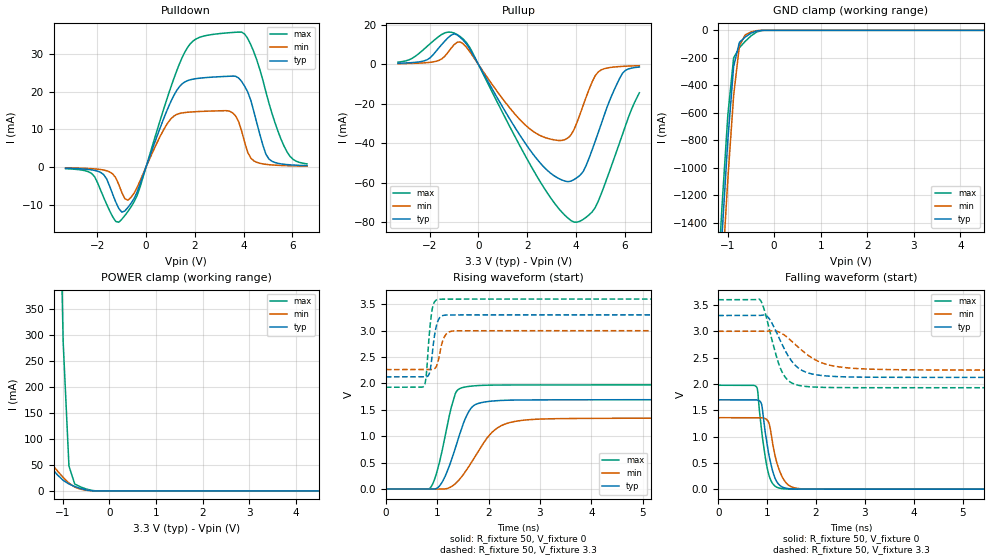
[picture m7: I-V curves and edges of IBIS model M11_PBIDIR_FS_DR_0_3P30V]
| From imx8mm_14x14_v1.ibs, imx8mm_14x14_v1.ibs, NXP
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[Model] M11_PBIDIR_FS_DR_0_3P30V
Model_type I/O
Vinl  =  0.54
Vinh  =  1.26
Vmeas =  0.9
| Capacitance   typ   min   max
C_comp   2.08161232969e-12   2.03493647009e-12   2.16777276051e-12
| Variables   typ   min   max
[GND Clamp Reference]   0   0   0
[POWER Clamp Reference]   3.3   3   3.6
[Pulldown Reference]   0   0   0
[Pullup Reference]   3.3   3   3.6
[Temperature Range]   25   125   -40
[Voltage Range]   3.3   3   3.6
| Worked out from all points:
|   slope of the pulldown table from 0 to 0.495 V, typ, clamps not added: 55.3 ohm
|   slope of the pullup table from 0 to 0.495 V, typ, clamps not added: 45.4 ohm
|   GND clamp passes 1 mA (typ) near -0.28 V on its own axis
|   POWER clamp passes 1 mA (typ) near -0.44 V on its own axis
|   falling waveform, R_fixture 50, V_fixture 0: 20-80 % time 192ps typ, 212ps min, 172ps max; typ from 1.7 V to 0 V
|   falling waveform, R_fixture 50, V_fixture 3.3: 20-80 % time 421ps typ, 641ps min, 303ps max; typ from 3.3 V to 2.12 V
|   rising waveform, R_fixture 50, V_fixture 0: 20-80 % time 361ps typ, 574ps min, 268ps max; typ from 0 V to 1.7 V
|   rising waveform, R_fixture 50, V_fixture 3.3: 20-80 % time 97.1ps typ, 110ps min, 84.1ps max; typ from 2.12 V to 3.3 V
[GND Clamp]
| Voltage   I(typ)   I(min)   I(max)
-3.3V     -15.63A    -15.86A    -15.46A
-1.241V   -2.232A    -2.527A    -2.015A
-1.117V   -1.487A    -1.785A    -1.276A
-993.1mV  -798.9mA   -1.083A    -616.8mA
-869mV    -263.4mA   -475.6mA   -200.8mA
-744.8mV  -87.36mA   -112.1mA   -126.1mA
-620.7mV  -49.17mA   -33.01mA   -80.34mA
-496.6mV  -20.8mA    -11.81mA   -40.7mA
-372.4mV  -3.877mA   -2.002mA   -11.64mA
-248.3mV  -117.5uA   -105.1uA   -542.9uA
6.6V      0A         0A         0A
[POWER Clamp]
| Voltage   I(typ)   I(min)   I(max)
-3.3V     11.6A      9.427A     14.09A
-1.862V   2.37A      558.5mA    4.855A
-1.738V   1.676A     202.6mA    4.157A
-1.614V   1.03A      99.77mA    3.468A
-1.49V    451mA      80.49mA    2.786A
-1.366V   91.11mA    66.06mA    2.111A
-1.241V   43.77mA    52.06mA    1.45A
-1.117V   30.97mA    38.55mA    817.5mA
-993.1mV  20.41mA    25.92mA    286.6mA
-869mV    13.37mA    15.08mA    47.85mA
-744.8mV  8.524mA    7.507mA    13.32mA
6.6V      0A         0A         0A
[Pulldown]
| Voltage   I(typ)   I(min)   I(max)
-3.3V     -336.6uA   -232.9uA   -466.4uA
-2.234V   -784.9uA   -464.4uA   -1.722mA
-1.738V   -2.046mA   -833.5uA   -8.118mA
-1.117V   -11.06mA   -4.708mA   -14.68mA
-620.7mV  -9.706mA   -8.13mA    -10.66mA
910.3mV   15.8mA     11.88mA    19.13mA
1.707V    22.93mA    14.52mA    31.79mA
3.797V    23.62mA    12.02mA    35.81mA
4.293V    17.72mA    2.358mA    32.49mA
5.038V    2.102mA    590.4uA    16.96mA
5.783V    618uA      327.6uA    3.967mA
6.6V      348.1uA    218.8uA    811.1uA
[Pullup]
| Voltage   I(typ)   I(min)   I(max)
-3.3V     583.1uA    366.4uA    1.137mA
-2.11V    2.303mA    895.4uA    9.049mA
-1.366V   11.98mA    4.309mA    16.03mA
-993.1mV  15.47mA    10.03mA    15.88mA
-620.7mV  12.26mA    10.41mA    12.81mA
2.162V    -44.15mA   -33.17mA   -51.6mA
3.3V      -57.84mA   -38.56mA   -73.11mA
3.921V    -58.36mA   -33.01mA   -79.87mA
4.293V    -54.37mA   -20.86mA   -78.55mA
4.914V    -34.57mA   -3.798mA   -69.37mA
5.907V    -4.528mA   -989.6uA   -35.53mA
6.6V      -1.319mA   -661.9uA   -14.37mA
[Ramp]
dV/dt_r   1.01838/0.360589n  0.81373/0.573821n  1.18486/0.268467n
dV/dt_f   0.70522/0.420856n  0.442179/0.64106n  1.0031/0.303181n
R_load = 50
[Falling Waveform]
R_fixture = 50
V_fixture = 0
V_fixture_min = 0
V_fixture_max = 0
| Time   V(typ)   V(min)   V(max)
0s        1.698V     1.359V     1.975V
783.8ps   1.697V     1.359V     1.944V
809.7ps   1.692V     1.359V     1.853V
891ps     1.601V     1.358V     1.091V
990.1ps   899.7mV    1.324V     459.2mV
1.07ns    507.8mV    1.128V     180.5mV
1.175ns   183.9mV    590.8mV    50.2mV
1.302ns   44.98mV    246.3mV    10.57mV
1.654ns   1.159mV    10.24mV    322.6uV
333.3ns   2.947uV    4.354uV    13.11uV
[Falling Waveform]
R_fixture = 50
V_fixture = 3.3
V_fixture_min = 3
V_fixture_max = 3.6
| Time   V(typ)   V(min)   V(max)
0s        3.3V       3V         3.6V
855ps     3.302V     3V         3.6V
930ps     3.312V     3.001V     3.448V
1.026ns   3.261V     3.003V     3.117V
1.247ns   2.87V      2.985V     2.36V
1.468ns   2.478V     2.841V     2.039V
1.846ns   2.207V     2.54V      1.947V
2.189ns   2.153V     2.379V     1.933V
2.663ns   2.133V     2.304V     1.929V
333.3ns   2.125V     2.263V     1.928V
[Rising Waveform]
R_fixture = 50
V_fixture = 0
V_fixture_min = 0
V_fixture_max = 0
| Time   V(typ)   V(min)   V(max)
0s        2.947uV    4.353uV    13.11uV
858.1ps   -1.64mV    -18.15uV   16.12mV
1.095ns   127mV      -3.305mV   721.2mV
1.262ns   507.3mV    35.87mV    1.501V
1.38ns    858.1mV    124.5mV    1.855V
1.682ns   1.557V     528mV      1.952V
2.253ns   1.678V     1.202V     1.97V
3.245ns   1.689V     1.331V     1.972V
10.4ns    1.693V     1.346V     1.974V
333.3ns   1.697V     1.356V     1.975V
[Rising Waveform]
R_fixture = 50
V_fixture = 3.3
V_fixture_min = 3
V_fixture_max = 3.6
| Time   V(typ)   V(min)   V(max)
0s        2.125V     2.263V     1.928V
742.9ps   2.124V     2.263V     1.952V
786ps     2.126V     2.263V     2.153V
849.2ps   2.197V     2.262V     2.978V
913.9ps   2.656V     2.267V     3.461V
1.008ns   3.173V     2.389V     3.591V
1.156ns   3.296V     2.911V     3.599V
1.349ns   3.299V     2.997V     3.599V
3.165ns   3.3V       3V         3.6V
333.3ns   3.3V       3V         3.6V
[Add Submodel]
| Submodel Name Mode
M11_PBIDIR_FS_DR_0_3P30V_T All
